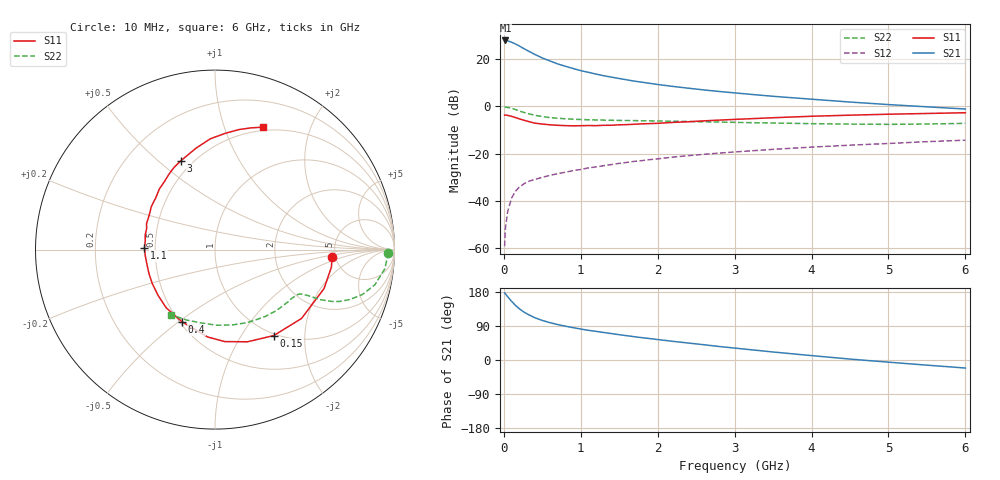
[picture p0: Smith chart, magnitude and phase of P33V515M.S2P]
! SIEMENS Small Signal Semiconductors
! BFP181
! Si NPN RF Bipolar Junction Transistor in SOT143
! VCE = 3.5 V  IC = 15 mA
! Common Emitter S-Parameters:  March  1996
# GHz  S  MA  R  50
!  f  S11  S21  S12  S22
! GHz  MAG  ANG  MAG  ANG  MAG  ANG  MAG  ANG
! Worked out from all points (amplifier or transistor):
!   36 points, 10 MHz to 6 GHz, reference 50 ohm
!   highest |S21| = 27.9 dB at 20 MHz (marker M1)
!   |S21| within 3 dB of that: start of sweep to 235.8 MHz
!   unconditionally stable (mu >= 1): 800 MHz to end of sweep
!   at 250 MHz: K = 0.46, MSG = 28.8 dB, |S12| = -33.0 dB
!   at 1.4 GHz: K = 1.20, MAG = 15.8 dB, |S12| = -24.6 dB
!   at 6 GHz: K = 1.01, MAG = 6.0 dB, |S12| = -14.3 dB
!   S11 on the Smith chart (normalised r, x): 10 MHz: 4.66, -0.70; 150 MHz: 0.97, -1.41; 400 MHz: 0.51, -0.52; 1.1 GHz: 0.44, +0.01; 3 GHz: 0.43, +0.59; 6 GHz: 0.46, +1.37
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0.01  0.6533 -3.8  24.83 177.1  0.0011 78.5  0.9634 -1.0
0.02  0.656 -8.5  24.85 174.9  0.0026 89.9  0.9616 -2.4
0.05  0.6451 -19.7  24.42 166.9  0.006 84.4  0.9521 -6.5
0.1  0.6161 -38.5  22.8 155.1  0.0114 71.3  0.9122 -12.4
0.15  0.5802 -55.6  20.99 144.3  0.0159 65.1  0.8591 -16.9
0.2  0.5446 -70.6  19.04 135.4  0.0195 61.4  0.8033 -20.2
0.25  0.5155 -83.9  17.05 128.0  0.0223 58.3  0.7543 -22.5
0.3  0.4884 -94.9  15.43 122.0  0.0252 55.3  0.7134 -23.9
0.4  0.4423 -114.5  12.66 111.8  0.0284 53.1  0.6499 -25.4
0.5  0.4232 -129.9  10.58 104.4  0.0315 51.4  0.608 -25.9
0.6  0.4072 -141.0  9.149 98.5  0.0347 51.9  0.5794 -26.3
0.7  0.3975 -151.6  7.916 93.5  0.0376 52.5  0.5606 -26.7
0.9  0.3881 -167.8  6.332 85.4  0.0437 53.0  0.5356 -27.5
1.1  0.393 178.5  5.249 78.3  0.0499 53.2  0.5213 -29.1
1.3  0.3974 168.1  4.445 72.5  0.0556 53.3  0.5122 -31.1
1.6  0.4113 154.4  3.645 64.1  0.0653 53.1  0.5029 -34.4
2.2  0.4582 132.6  2.644 49.2  0.0845 50.5  0.4846 -43.0
3  0.5301 111.1  1.929 31.5  0.1085 45.4  0.4583 -56.6
3.5  0.5749 100.6  1.634 21.1  0.1233 41.9  0.4445 -66.3
4.5  0.6516 84.7  1.235 2.4  0.1509 33.8  0.4215 -88.7
5.5  0.7078 73.4  0.979 -13.6  0.1792 26.5  0.4235 -112.2
6  0.734 68.4  0.879 -21.2  0.1926 22.3  0.437 -124.0
